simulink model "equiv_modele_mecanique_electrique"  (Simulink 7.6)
settings: Solver=ode15s  StartTime=0.0  StopTime=0.001  RelTol=1e-3
InitFcn:
  | clc
  | clear all
  | J=0.1;
  | f=10;
  | k=0.01;
  | F=1;
StopFcn:
  | clc
  | load equiv_meca_elec.mat
  | plot(x(1,:),x(2,:),x(1,:),x(3,:))
  | title('Réponse indicielle des circuits, mécanique et électrique, équivalents')
  | grid
  | xlabel('temps')
libraries: fl_lib x11, nesl_utility x6

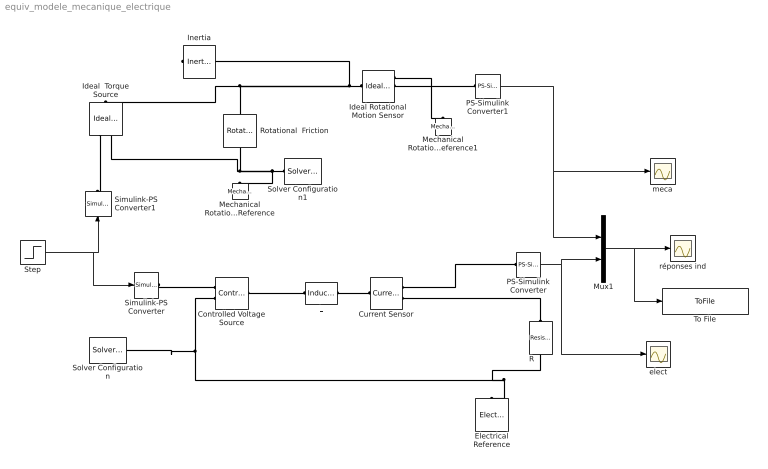
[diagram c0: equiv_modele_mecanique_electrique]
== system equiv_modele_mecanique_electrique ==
  Controlled Voltage Source : fl_lib/Electrical/Electrical Sources/Controlled Voltage Source  DialogController=NetworkEngine.DynNeDlgSource  SystemSampleTime=-1  i_Log=off  v_Log=off  LocalVarNames=|i|v  LocalVarDescs=|i|v  LocalVarLogging=[0 0]
  Current Sensor : fl_lib/Electrical/Electrical Sensors/Current Sensor  DialogController=NetworkEngine.DynNeDlgSource  SystemSampleTime=-1  i1_Log=off  v1_Log=off  LocalVarNames=|i1|v1  LocalVarDescs=|i1|v1  LocalVarLogging=[0 0]
  Electrical Reference : fl_lib/Electrical/Electrical Elements/Electrical Reference  DialogController=NetworkEngine.DynNeDlgSource  SystemSampleTime=-1  i_Log=off  LocalVarNames=|i  LocalVarDescs=|i  LocalVarLogging=0
  Ideal  Torque Source : fl_lib/Mechanical/Mechanical Sources/Ideal Torque Source  DialogController=NetworkEngine.DynNeDlgSource  SystemSampleTime=-1  w_Log=off  t_Log=off  LocalVarNames=|w|t  LocalVarDescs=|w|t  LocalVarLogging=[0 0]
  Ideal Rotational Motion Sensor : fl_lib/Mechanical/Mechanical Sensors/Ideal Rotational Motion Sensor  DialogController=NetworkEngine.DynNeDlgSource  SystemSampleTime=-1  offset=0 rad  w_Log=off  t_Log=off  phi_Log=off  LocalVarNames=|w|t|phi  LocalVarDescs=|w|t|phi  LocalVarLogging=[0 0 0]
  Inertia : fl_lib/Mechanical/Rotational Elements/Inertia  DialogController=NetworkEngine.DynNeDlgSource  SystemSampleTime=-1  inertia=0.01 kg*m^2  initial_velocity=0 rad/s  t_Log=off  LocalVarNames=|t  LocalVarDescs=|t  LocalVarLogging=0
  L : fl_lib/Electrical/Electrical Elements/Inductor  DialogController=NetworkEngine.DynNeDlgSource  SystemSampleTime=-1  l=1e-2 H  i0=0 A  r=0 Ohm  g=1e-9 1/Ohm  i_Log=off  v_Log=off  i_L_Log=off  LocalVarNames=|i|v|i_L  LocalVarDescs=|i|v|Internal variable for current through inductor term  LocalVarLogging=[0 0 0]
  Mechanical Rotational Reference : fl_lib/Mechanical/Rotational Elements/Mechanical Rotational Reference  DialogController=NetworkEngine.DynNeDlgSource  SystemSampleTime=-1  t_Log=off  LocalVarNames=|t  LocalVarDescs=|t  LocalVarLogging=0
  Mechanical Rotational Reference1 : fl_lib/Mechanical/Rotational Elements/Mechanical Rotational Reference  DialogController=NetworkEngine.DynNeDlgSource  SystemSampleTime=-1  t_Log=off  LocalVarNames=|t  LocalVarDescs=|t  LocalVarLogging=0
  Mux1 : Mux  Inputs=2
  PS-Simulink Converter : nesl_utility/PS-Simulink Converter  DialogController=NetworkEngine.DynNeUtilDlgSource  SystemSampleTime=-1  PhysicalDomain=network_engine_domain  LeftPortType=input  RightPortType=output  SubClassName=ps_output  Unit=1  AffineConversion=off
  PS-Simulink Converter1 : nesl_utility/PS-Simulink Converter  DialogController=NetworkEngine.DynNeUtilDlgSource  SystemSampleTime=-1  PhysicalDomain=network_engine_domain  LeftPortType=input  RightPortType=output  SubClassName=ps_output  Unit=1  AffineConversion=off
  R : fl_lib/Electrical/Electrical Elements/Resistor  DialogController=NetworkEngine.DynNeDlgSource  SystemSampleTime=-1  R=0.1 kOhm  i_Log=off  v_Log=off  LocalVarNames=|i|v  LocalVarDescs=|i|v  LocalVarLogging=[0 0]
  Rotational  Friction : fl_lib/Mechanical/Rotational Elements/Rotational Friction  DialogController=NetworkEngine.DynNeDlgSource  SystemSampleTime=-1  brkwy_trq=0.001 N*m  Col_trq=0.00001 N*m  visc_coef=100 N*m/(rad/s)  trans_coef=10 s/rad  vel_thr=1e-4 rad/s  t_Log=off  w_Log=off  LocalVarNames=|t|w  LocalVarDescs=|t|w  LocalVarLogging=[0 0]
  Simulink-PS Converter : nesl_utility/Simulink-PS Converter  DialogController=NetworkEngine.DynNeUtilDlgSource  SystemSampleTime=-1  PhysicalDomain=network_engine_domain  LeftPortType=input  RightPortType=output  SubClassName=ps_input  Unit=1  AffineConversion=off  InputFilterTimeConstant=.001  UdotUserProvided=0
  Simulink-PS Converter1 : nesl_utility/Simulink-PS Converter  DialogController=NetworkEngine.DynNeUtilDlgSource  SystemSampleTime=-1  PhysicalDomain=network_engine_domain  LeftPortType=input  RightPortType=output  SubClassName=ps_input  Unit=1  AffineConversion=off  InputFilterTimeConstant=.001  UdotUserProvided=0
  Solver Configuration : nesl_utility/Solver Configuration  DialogController=NetworkEngine.DynNeUtilDlgSource  SystemSampleTime=-1  PhysicalDomain=network_engine_domain  LeftPortType=input  RightPortType=generic  SubClassName=solver  Accelerate=off  Profile=off  ResidualTolerance=1e-9  MaxNonlinIter=3  MaxModeIter=2  DoFixedCost=off  UseLocalSampling=off  DoDC=off  LinearAlgebra=Sparse  LocalSolverSampleTime=.001  LocalSolverChoice=NE_BACKWARD_EULER_ADVANCER  UseLocalSolver=off
  Solver Configuration1 : nesl_utility/Solver Configuration  DialogController=NetworkEngine.DynNeUtilDlgSource  SystemSampleTime=-1  PhysicalDomain=network_engine_domain  LeftPortType=input  RightPortType=generic  SubClassName=solver  Accelerate=off  Profile=off  ResidualTolerance=1e-9  MaxNonlinIter=3  MaxModeIter=2  DoFixedCost=off  UseLocalSampling=off  DoDC=off  LinearAlgebra=Sparse  LocalSolverSampleTime=.001  LocalSolverChoice=NE_BACKWARD_EULER_ADVANCER  UseLocalSolver=off
  Step : Step  Time=0.0002  After=F  SampleTime=0
  To File : ToFile  Filename=equiv_meca_elec  MatrixName=x
  elect : Scope
  meca : Scope
  réponses ind : Scope
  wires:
  PS-Simulink Converter/1 -> Mux1/2, elect/1
  PS-Simulink Converter1/1 -> Mux1/1, meca/1
  Step/1 -> Simulink-PS Converter1/1, Simulink-PS Converter/1
  Mux1/1 -> réponses ind/1, To File/1
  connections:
  R/LConn1 -- Current Sensor/RConn2
  L/RConn1 -- Current Sensor/LConn1
  Current Sensor/RConn1 -- PS-Simulink Converter/LConn1
  Controlled Voltage Source/LConn1 -- L/LConn1
  Controlled Voltage Source/RConn2 -- Electrical Reference/LConn1 -- R/RConn1 -- Solver Configuration/RConn1
  Simulink-PS Converter/RConn1 -- Controlled Voltage Source/RConn1
  PS-Simulink Converter1/LConn1 -- Ideal Rotational Motion Sensor/RConn2
  Ideal Rotational Motion Sensor/LConn1 -- Rotational  Friction/LConn1 -- Ideal  Torque Source/LConn1 -- Inertia/LConn1
  Ideal  Torque Source/RConn1 -- Simulink-PS Converter1/RConn1
  Solver Configuration1/RConn1 -- Rotational  Friction/RConn1 -- Mechanical Rotational Reference/LConn1 -- Ideal  Torque Source/RConn2
  Ideal Rotational Motion Sensor/RConn1 -- Mechanical Rotational Reference1/LConn1
